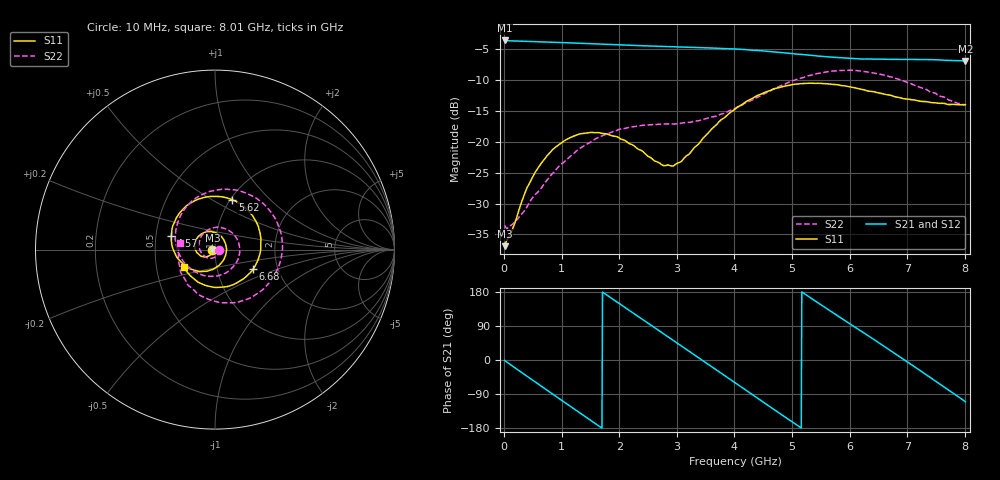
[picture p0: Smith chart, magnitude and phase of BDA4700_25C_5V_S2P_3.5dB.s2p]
!Agilent Technologies,E5071B,MY42404982,A.09.10
!Date: Mon Oct 20 13:27:39 2025
!Data & Calibration Information:
!Freq	S11:SOLT2(ON)	S21:SOLT2(ON)	S12:SOLT2(ON)	S22:SOLT2(ON)
# Hz S RI R 50
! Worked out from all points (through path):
!   801 points, 10 MHz to 8.01 GHz, reference 50 ohm
!   highest |S21| = -3.62 dB at 10 MHz (marker M1); lowest = -6.9 dB at 8.01 GHz (marker M2)
!   group delay of S21, straight-line fit = 287 ps
!   lowest |S11| = -36.9 dB at 10 MHz (marker M3), VSWR 1.03, Z = 48.6 - j0.153 ohm
!   |S11| at or under -10 dB: start of sweep to end of sweep
!   |S22| runs from -34.0 to -8.4 dB; largest |S21 - S12| = 0.0051
!   S11 on the Smith chart (normalised r, x): 10 MHz: 0.97, -0.00; 4.57 GHz: 0.60, +0.10; 5.62 GHz: 1.02, +0.62; 6.68 GHz: 1.49, -0.35; 8.01 GHz: 0.69, -0.14
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1e7  -0.0142 -0.00158  0.6594 -0.0142  0.6593 -0.0149  0.021 -0.00184
3.3e8  -0.0233 -0.0263  0.5288 -0.3774  0.5286 -0.3779  0.0191 -0.0187
7.2e8  -0.0621 -0.0405  0.146 -0.624  0.1461 -0.6241  -0.00952 -0.0463
1.02e9  -0.0977 -0.0204  -0.2 -0.6011  -0.2003 -0.6015  -0.0544 -0.0396
1.35e9  -0.113 0.0275  -0.4998 -0.3756  -0.5004 -0.3756  -0.0889 0.0154
1.63e9  -0.0948 0.0711  -0.6125 -0.0815  -0.6129 -0.0814  -0.0733 0.0789
1.92e9  -0.0516 0.098  -0.5631 0.2356  -0.5632 0.2355  -0.00898 0.1215
2.32e9  0.0177 0.0858  -0.2612 0.54  -0.261 0.5402  0.099 0.0903
2.68e9  0.0583 0.0347  0.117 0.5807  0.1173 0.5808  0.1379 -0.011
3.06e9  0.0554 -0.0404  0.4539 0.369  0.4518 0.3708  0.0854 -0.112
3.36e9  0.0151 -0.093  0.573 0.0821  0.5736 0.0811  0.00317 -0.1477
3.67e9  -0.0588 -0.1214  0.521 -0.2338  0.521 -0.2354  -0.0892 -0.1335
4.01e9  -0.1556 -0.0972  0.2833 -0.4857  0.2837 -0.4856  -0.1728 -0.0701
4.57e9  -0.244 0.0746  -0.2568 -0.4743  -0.2562 -0.4748  -0.2124 0.1331
4.97e9  -0.1771 0.2262  -0.4868 -0.1781  -0.4873 -0.1794  -0.106 0.2872
5.35e9  -0.0262 0.2959  -0.4724 0.1606  -0.4734 0.1597  0.0938 0.3341
5.62e9  0.097 0.2777  -0.3381 0.3499  -0.3379 0.3505  0.2406 0.2789
6.13e9  0.2458 0.112  0.0566 0.4655  0.0592 0.4661  0.3763 0.0105
6.68e9  0.2121 -0.1099  0.4104 0.2169  0.4113 0.2163  0.2216 -0.2541
7.24e9  0.0338 -0.2096  0.4034 -0.2281  0.4026 -0.2288  -0.0585 -0.2671
7.63e9  -0.0942 -0.1817  0.1549 -0.4298  0.1537 -0.4307  -0.1882 -0.1333
8.01e9  -0.1753 -0.0949  -0.1548 -0.4226  -0.1548 -0.4232  -0.1954 0.0383
